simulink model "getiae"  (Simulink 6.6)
settings: Solver=ode23s  StartTime=0.0  StopTime=400  RelTol=1e-6
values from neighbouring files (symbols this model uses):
  design = []    [designpid.m]
libraries: simulink x2, cstextras x2, cstblocks x1

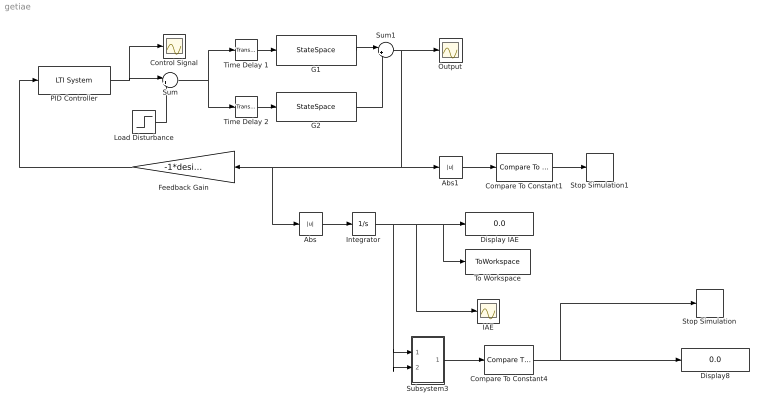
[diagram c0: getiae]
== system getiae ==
  Abs : Abs
  Abs1 : Abs
  Compare To Constant1 : simulink/Logic and Bit Operations/Compare To Constant  SystemSampleTime=-1  relop=>  const=5e12  LogicOutDataTypeMode=boolean  ZeroCross=off
  Compare To Constant4 : simulink/Logic and Bit Operations/Compare To Constant  SystemSampleTime=-1  relop=<=  const=0.001  LogicOutDataTypeMode=boolean  ZeroCross=off
  Control Signal : Scope
  Display IAE : Display
  Display8 : Display
  Feedback Gain : Gain  Orientation=left  Gain=-1*design.sim.sgn
  G1 : StateSpace  A=design.sim.G1a  B=design.sim.G1b  C=design.sim.G1c  D=design.sim.G1d
  G2 : StateSpace  A=design.sim.G2a  B=design.sim.G2b  C=design.sim.G2c  D=design.sim.G2d
  IAE : Scope
  Integrator : Integrator
  Load Disturbance : Step  Time=0  SampleTime=0
  Output : Scope
  PID Controller : cstblocks/LTI System  SystemSampleTime=-1  sys=design.PID.Gr  IC=[]
  Stop Simulation : Stop
  Stop Simulation1 : Stop
  Subsystem3 : Subsystem
  Sum : Sum  Inputs=|++
  Sum1 : Sum  Inputs=|++
  Time Delay 1 : cstextras/Transport Delay (masked)  Tag=InputDelayBlock  SystemSampleTime=-1  Td=design.sim.L1  u0=0  bufsize=100000
  Time Delay 2 : cstextras/Transport Delay (masked)  Tag=InputDelayBlock  SystemSampleTime=-1  Td=design.sim.L2  u0=0  bufsize=100000
  To Workspace : ToWorkspace  VariableName=IAE_val  SampleTime=-1  SaveFormat=Array
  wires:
  Sum/1 -> Time Delay 1/1, Time Delay 2/1
  PID Controller/1 -> Sum/1, Control Signal/1
  Load Disturbance/1 -> Sum/2
  Time Delay 1/1 -> G1/1
  G1/1 -> Sum1/1
  Time Delay 2/1 -> G2/1
  Sum1/1 -> Output/1, Feedback Gain/1, Abs/1, Abs1/1
  Feedback Gain/1 -> PID Controller/1
  G2/1 -> Sum1/2
  Integrator/1 -> To Workspace/1, Display IAE/1, IAE/1, Subsystem3/1(In1), Subsystem3/2(In2)
  Subsystem3/1(Out1) -> Compare To Constant4/1
  Compare To Constant4/1 -> Display8/1, Stop Simulation/1
  Abs/1 -> Integrator/1
  Abs1/1 -> Compare To Constant1/1
  Compare To Constant1/1 -> Stop Simulation1/1

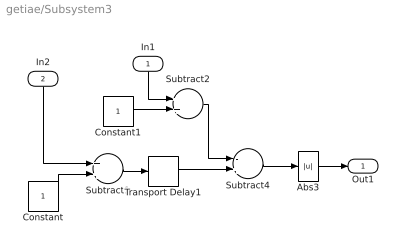
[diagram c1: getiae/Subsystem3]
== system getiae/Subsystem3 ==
  In1 : Inport  Orientation=down
  In2 : Inport  Orientation=down  Port=2
  Abs3 : Abs  ZeroCross=off
  Constant : Constant
  Constant1 : Constant
  Subtract1 : Sum  OutScaling=2^-10
  Subtract2 : Sum  OutScaling=2^-10
  Subtract4 : Sum  Inputs=-+  OutScaling=2^-10
  Transport Delay1 : TransportDelay  DelayTime=25  BufferSize=100000
  Out1 : Outport
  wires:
  Abs3/1 -> Out1/1
  Subtract4/1 -> Abs3/1
  Transport Delay1/1 -> Subtract4/2
  Constant/1 -> Subtract1/2
  In2/1 -> Subtract1/1
  Subtract1/1 -> Transport Delay1/1
  Constant1/1 -> Subtract2/2
  Subtract2/1 -> Subtract4/1
  In1/1 -> Subtract2/1
